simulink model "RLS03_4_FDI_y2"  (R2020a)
settings: Solver=ode45  StartTime=0.0  StopTime=100  RelTol=1e-3  EnableMultiTasking=on
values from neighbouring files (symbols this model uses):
  Ts = 0.05    [init_model.m]
libraries: ctrlSharedLib x1

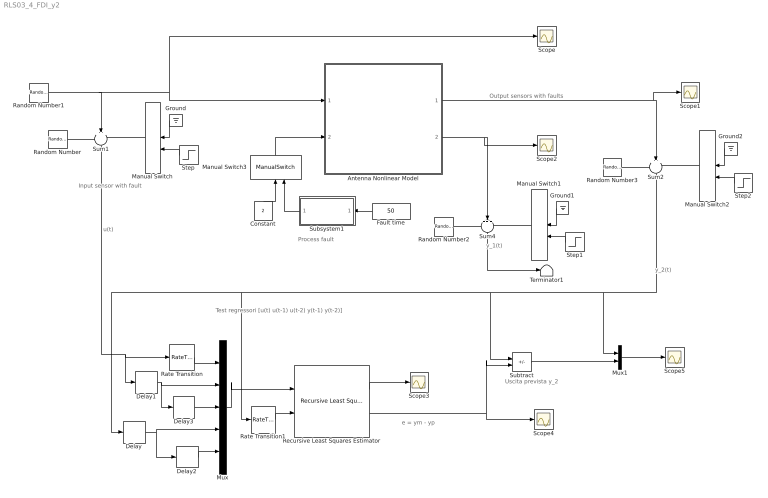
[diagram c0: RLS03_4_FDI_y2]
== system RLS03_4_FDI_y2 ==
  note: Uscita prevista y_2
  note: e = ym - yp
  note: Test regressori [u(t) u(t-1) u(t-2) y(t-1) y(t-2)]
  note: u(t)
  note: Output sensors with faults
  note: Process fault
  note: Input sensor with fault
  note: y_1(t)
  note: y_2(t)
  Antenna Nonlinear Model : Subsystem
  Constant : Constant  Value=2
  Delay{,1..3} (4 alike) : Delay  DelayLength=1  SampleTime=Ts
  Fault time : Constant  Value=50
  Ground : Ground
  Ground1 : Ground
  Ground2 : Ground
  Manual Switch : ManualSwitch
  Manual Switch1 : ManualSwitch
  Manual Switch2 : ManualSwitch
  Manual Switch3 : ManualSwitch  CurrentSetting=0
  Mux : Mux  Inputs=5
  Mux1 : Mux  Inputs=2
  Random Number : RandomNumber  Variance=0.0001  Seed=1  SampleTime=Ts
  Random Number1 : RandomNumber  Variance=0.1  SampleTime=10
  Random Number2 : RandomNumber  Variance=0.00001  Seed=2  SampleTime=Ts
  Random Number3 : RandomNumber  Variance=0.00001  Seed=3  SampleTime=Ts
  Rate Transition : RateTransition  OutPortSampleTime=Ts
  Rate Transition1 : RateTransition  OutPortSampleTime=Ts
  Recursive Least Squares Estimator : ctrlSharedLib/Recursive Least Squares Estimator  InitialEstimateSource=None  InitialParameterData=5  P0=1e4  InitialRegressors=0  InitialOutputs=0  History=Infinite  WindowLength=200  EstimationMethod=Forgetting Factor  AdaptationParameter=0.97  HasTimeVaryingAdaptationParameter=off  NormalizationBias=eps  OutputError=on  OutputP=off  AddEnablePort=off  InputProcessing=Sample-based  Ts=Ts
  Scope{,1..5} (6 alike) : Scope
  Step : Step  Time=50  SampleTime=0
  Step1 : Step  Time=1500  SampleTime=0
  Step2 : Step  Time=50  SampleTime=0
  Subsystem1 : Subsystem
  Subtract : Sum  Inputs=+-
  Sum1 : Sum  Inputs=+++  SaturateOnIntegerOverflow=on
  Sum2 : Sum  Inputs=+++  SaturateOnIntegerOverflow=on
  Sum4 : Sum  Inputs=+++  SaturateOnIntegerOverflow=on
  Terminator1 : Terminator
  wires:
  Random Number1/1 -> Scope/1, Antenna Nonlinear Model/1(force), Sum1/2
  Random Number/1 -> Sum1/1
  Manual Switch/1 -> Sum1/3
  Sum1/1 -> Rate Transition/1, Delay1/1
  Ground/1 -> Manual Switch/1
  Step/1 -> Manual Switch/2
  Random Number2/1 -> Sum4/1
  Sum4/1 -> Terminator1/1
  Ground1/1 -> Manual Switch1/1
  Manual Switch1/1 -> Sum4/3
  Step1/1 -> Manual Switch1/2
  Antenna Nonlinear Model/2(velocity) -> Sum4/2, Scope2/1
  Random Number3/1 -> Sum2/1
  Ground2/1 -> Manual Switch2/1
  Manual Switch2/1 -> Sum2/3
  Step2/1 -> Manual Switch2/2
  Antenna Nonlinear Model/1(angle) -> Sum2/2, Scope1/1
  Sum2/1 -> Mux1/1, Subtract/1, Rate Transition1/1, Delay/1
  Fault time/1 -> Subsystem1/1(Fault time)
  Subsystem1/1(Fault) -> Manual Switch3/2
  Manual Switch3/1 -> Antenna Nonlinear Model/2(drag)
  Constant/1 -> Manual Switch3/1
  Mux/1 -> Recursive Least Squares Estimator/1
  Rate Transition1/1 -> Recursive Least Squares Estimator/2
  Recursive Least Squares Estimator/1 -> Scope3/1
  Recursive Least Squares Estimator/2 -> Scope4/1, Subtract/2
  Subtract/1 -> Mux1/2
  Mux1/1 -> Scope5/1
  Rate Transition/1 -> Mux/1
  Delay1/1 -> Delay3/1, Mux/2
  Delay/1 -> Delay2/1, Mux/4
  Delay2/1 -> Mux/5
  Delay3/1 -> Mux/3

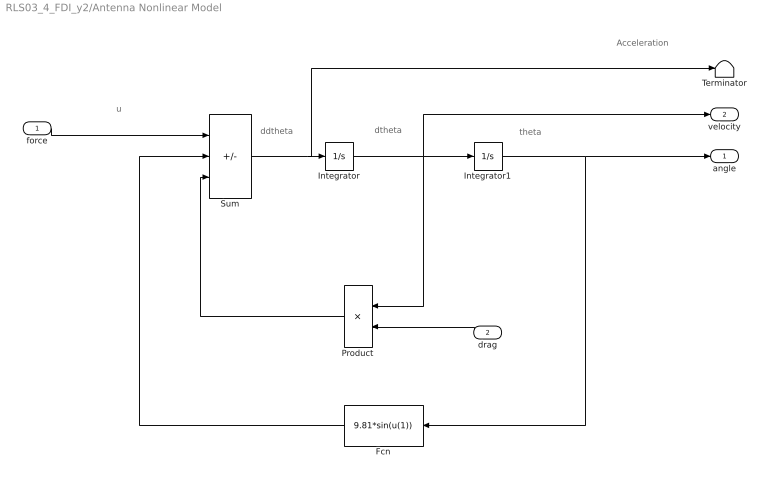
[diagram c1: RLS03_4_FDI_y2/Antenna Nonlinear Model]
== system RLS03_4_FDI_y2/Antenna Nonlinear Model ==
  note: Acceleration
  note: ddtheta
  note: dtheta
  note: theta
  note: u
  force : Inport
  drag : Inport  Port=2
  Fcn : Fcn  Expr=9.81*sin(u(1))
  Integrator : Integrator
  Integrator1 : Integrator  InitialCondition=(pi/180)*90
  Product : Product
  Sum : Sum  Inputs=+--  SaturateOnIntegerOverflow=on
  Terminator : Terminator
  angle : Outport
  velocity : Outport  Port=2
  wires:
  Sum/1 -> Terminator/1, Integrator/1
  Integrator/1 -> Product/1, Integrator1/1, velocity/1
  Integrator1/1 -> angle/1, Fcn/1
  Fcn/1 -> Sum/2
  Product/1 -> Sum/3
  force/1 -> Sum/1
  drag/1 -> Product/2

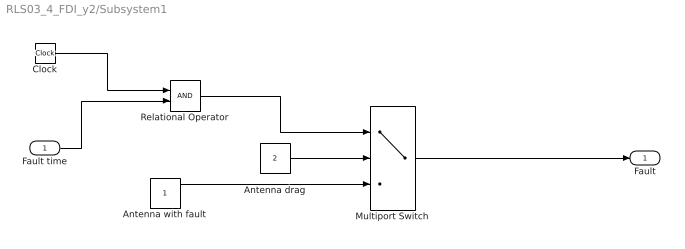
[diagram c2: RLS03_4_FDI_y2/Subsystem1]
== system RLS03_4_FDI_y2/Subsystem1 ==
  Fault time : Inport
  Antenna drag : Constant  Value=2
  Antenna with fault : Constant
  Clock : Clock
  Multiport Switch : MultiPortSwitch  DataPortOrder=Zero-based contiguous  Inputs=2  zeroidx=on
  Relational Operator : RelationalOperator  OutDataTypeStr=boolean  RndMeth=Simplest
  Fault : Outport
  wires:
  Clock/1 -> Relational Operator/1
  Fault time/1 -> Relational Operator/2
  Antenna drag/1 -> Multiport Switch/2
  Relational Operator/1 -> Multiport Switch/1
  Multiport Switch/1 -> Fault/1
  Antenna with fault/1 -> Multiport Switch/3
